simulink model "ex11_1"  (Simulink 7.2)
settings: Solver=ode45  StartTime=0.0  StopTime=10.0  RelTol=1e-3

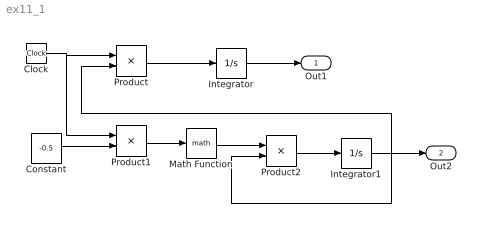
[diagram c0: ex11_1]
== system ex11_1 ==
  Clock : Clock
  Constant : Constant  Value=-0.5  OutDataType=sfix(16)  OutScaling=2^0
  Integrator : Integrator
  Integrator1 : Integrator
  Math Function : Math  OutDataType=sfix(16)  OutScaling=2^0
  Product : Product  OutDataType=sfix(16)  OutScaling=2^0
  Product1 : Product  OutDataType=sfix(16)  OutScaling=2^0
  Product2 : Product  OutDataType=sfix(16)  OutScaling=2^0
  Out1 : Outport  OutDataType=sfix(16)  OutScaling=2^0
  Out2 : Outport  Port=2  OutDataType=sfix(16)  OutScaling=2^0
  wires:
  Clock/1 -> Product/1, Product1/1
  Product/1 -> Integrator/1
  Integrator/1 -> Out1/1
  Constant/1 -> Product1/2
  Product1/1 -> Math Function/1
  Math Function/1 -> Product2/1
  Product2/1 -> Integrator1/1
  Integrator1/1 -> Out2/1, Product2/2, Product/2
